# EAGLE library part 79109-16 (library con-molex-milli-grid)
RECEPTACAL
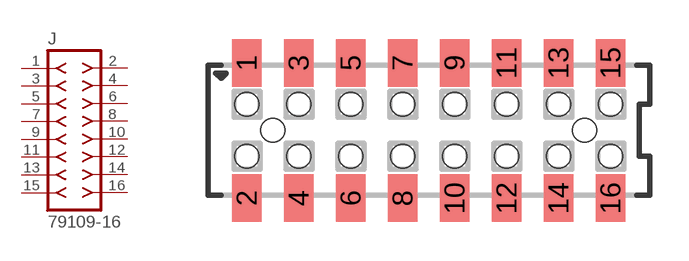
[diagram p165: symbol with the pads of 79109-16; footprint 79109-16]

Designator prefix J

## 79109-16  [79109-16]
1  1  pas
2  2  pas
3  3  pas
4  4  pas
5  5  pas
6  6  pas
7  7  pas
8  8  pas
9  9  pas
10  10  pas
11  11  pas
12  12  pas
13  13  pas
14  14  pas
15  15  pas
16  16  pas

## Footprint 79109-16 (pad centres in mm)
RECEPTACAL SMD Dual Row, Vertical, Pass-Thru
smd 1.12 x 1.83: 1 -7,2.6; 2 -7,-2.6; 3 -5,2.6; 4 -5,-2.6; 5 -3,2.6; 6 -3,-2.6; 7 -1,2.6; 8 -1,-2.6; 9 1,2.6; 10 1,-2.6; 11 3,2.6; 12 3,-2.6; 13 5,2.6; 14 5,-2.6; 15 7,2.6; 16 7,-2.6
hole 0.914 at -6,0
hole 0.914 at -7,1
hole 0.914 at -7,-1
hole 0.914 at -5,-1
hole 0.914 at -5,1
hole 0.914 at -3,-1
hole 0.914 at -3,1
hole 0.914 at 6,0
hole 0.914 at -1,1
hole 0.914 at -1,-1
hole 0.914 at 1,1
hole 0.914 at 1,-1
hole 0.914 at 3,1
hole 0.914 at 3,-1
hole 0.914 at 5,1
hole 0.914 at 5,-1
hole 0.914 at 7,-1
hole 0.914 at 7,1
